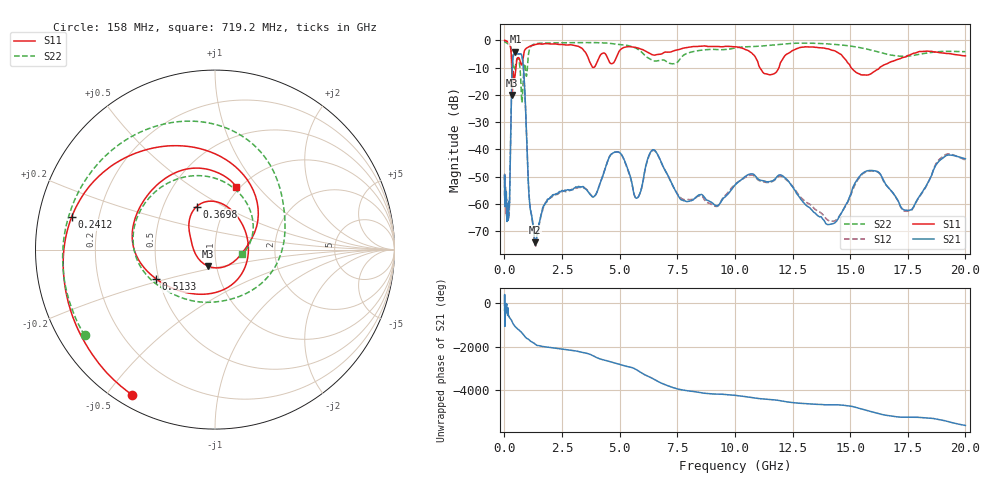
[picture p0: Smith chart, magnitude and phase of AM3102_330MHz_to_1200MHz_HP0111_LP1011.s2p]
! Date/Time: Tue, Sep 11, 2018 5:16 PM
! Network Analyzer: Agilent Technologies E8362B Rev: A.07.50.63
! Sweep from 0.010 to 20.000 GHz, 1601 Points, Sweep Type: LOG
! Power Supply: 4.949 V, 0.001 A
# Hz S DB R 50
!freq MagS11 AngS11 MagS21 AngS21 MagS12 AngS12 MagS22 AngS22
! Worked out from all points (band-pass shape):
!   1601 points, 10 MHz to 20 GHz, reference 50 ohm
!   highest |S21| = -4.06 dB at 480.2 MHz (marker M1); lowest = -74.1 dB at 1.334 GHz (marker M2)
!   |S21| within 3 dB of the highest: 364.5 MHz to 790.8 MHz (426.3 MHz wide, 73.8 % of centre)
!   lowest |S11| = -20.0 dB at 341.1 MHz (marker M3), VSWR 1.22, Z = 45.3 - j8.33 ohm
!   |S11| at or under -10 dB: 317.3 MHz to 499.4 MHz (182.1 MHz wide, 44.6 % of centre); 11.08 GHz to 11.91 GHz (828.2 MHz wide, 7.2 % of centre); 15.04 GHz to 16.28 GHz (1.239 GHz wide, 7.91 % of centre)
!   |S22| runs from -22.8 to -0.3 dB; largest |S21 - S12| = 0.011
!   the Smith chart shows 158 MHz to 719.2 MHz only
!   S11 on the Smith chart (normalised r, x): 158 MHz: 0.05, -0.58; 241.2 MHz: 0.10, +0.11; 369.8 MHz: 0.73, +0.38; 513.3 MHz: 0.48, -0.18; 719.2 MHz: 0.96, +0.77
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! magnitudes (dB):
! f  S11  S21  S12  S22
! 10 MHz  0.0  -51.7  -49.1  -0.3
! 35.55 MHz  0.0  -58.4  -57.8  -0.5
! 126.4 MHz  -0.4  -64.5  -64.0  -1.1
! 158 MHz  -0.6  -65.1  -64.5  -1.2
! 241.2 MHz  -1.7  -51.7  -52.6  -1.8
! 341.1 MHz  -20.0  -9.8  -9.9  -6.4
! 369.8 MHz  -11.7  -6.7  -6.8  -8.5
! 447.2 MHz  -13.8  -4.2  -4.2  -10.4
! 480.2 MHz  -11.7  -4.1  -4.1  -9.3
! 513.3 MHz  -8.7  -4.2  -4.4  -7.8
! 719.2 MHz  -8.7  -4.9  -5.0  -16.2
! 849.3 MHz  -4.5  -12.9  -13.0  -9.8
! 1.334 GHz  -1.5  -74.1  -75.1  -1.3
! 1.59 GHz  -1.3  -64.0  -64.1  -1.0
! 3.884 GHz  -9.9  -57.3  -57.4  -0.8
! 4.809 GHz  -7.2  -41.0  -41.0  -1.3
! 5.652 GHz  -2.5  -57.1  -57.1  -2.6
! 6.487 GHz  -5.4  -40.1  -40.3  -7.5
! 7.808 GHz  -2.8  -58.8  -58.4  -5.2
! 11.92 GHz  -9.9  -49.4  -49.9  -1.5
! 14.07 GHz  -3.1  -67.6  -66.1  -1.3
! 20 GHz  -5.7  -43.4  -44.0  -4.1
